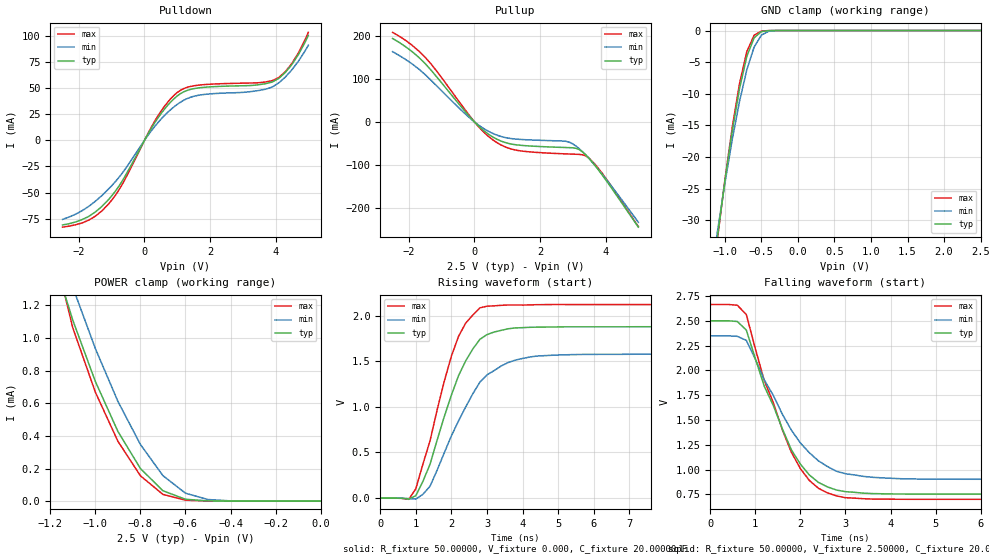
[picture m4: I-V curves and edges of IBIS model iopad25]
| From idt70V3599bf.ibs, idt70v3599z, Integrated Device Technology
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|   Model iopad25
[Model]   iopad25
Model_type   I/O
Polarity   Non-Inverting
Enable   Active-Low
Vinl =  0.70000V
Vinh =  1.70000V
Vmeas =  1.25000V
C_comp   4.50000pF   NA   NA
[Temperature Range]   25.00000   100.00000   0.000
[Voltage Range]   2.50000V   2.30000V   2.70000V
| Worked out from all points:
|   slope of the pulldown table from 0 to 0.375 V, typ, clamps not added: 19 ohm
|   slope of the pullup table from 0 to 0.375 V, typ, clamps not added: 14.7 ohm
|   GND clamp passes 1 mA (typ) near -0.58 V on its own axis
|   POWER clamp passes 1 mA (typ) near -1.07 V on its own axis
|   rising waveform, R_fixture 50.00000, V_fixture 0.000, C_fixture 20.00000pF: 20-80 % time 997ps typ, 1.18ns min, 891ps max; typ from 0 V to 1.88 V
|   falling waveform, R_fixture 50.00000, V_fixture 2.50000, C_fixture 20.00000pF: 20-80 % time 957ps typ, 1.1ns min, 930ps max; typ from 2.5 V to 0.752 V
[Pulldown]
| voltage   I(typ)   I(min)   I(max)
-2.5V     -80.9mA    -75.6mA    -83mA
-1.7V     -72.72mA   -63.11mA   -76.3mA
-1.1V     -56.75mA   -46.65mA   -61mA
-700mV    -39.93mA   -32.22mA   -43.24mA
400mV     20.93mA    16.57mA    22.86mA
1V        42.48mA    34.41mA    45.78mA
1.6V      49.93mA    42.82mA    52.59mA
3.2V      52.4mA     46.46mA    54.8mA
3.9V      55.8mA     51.01mA    57.1mA
4.1V      59.27mA    54.98mA    60.15mA
4.5V      72.61mA    67.54mA    73.61mA
5V        100.4mA    90.94mA    103.3mA
[Pullup]
| voltage   I(typ)   I(min)   I(max)
-2.5V     193.7mA    163.2mA    208mA
-1.9V     162.9mA    134.5mA    177.7mA
-1.5V     135.1mA    109.5mA    149.5mA
0V        0A         0A         0A
600mV     -36.73mA   -28.02mA   -43.74mA
900mV     -46.86mA   -35.51mA   -56.68mA
1.3V      -53.27mA   -39.97mA   -65.84mA
2.8V      -59.36mA   -45.06mA   -74.12mA
3.1V      -61.19mA   -56.09mA   -74.96mA
3.4V      -76.58mA   -76.99mA   -79.01mA
3.7V      -103mA     -102.7mA   -99.96mA
5V        -244.1mA   -232.8mA   -243mA
[GND_clamp]
| voltage   I(typ)   I(min)   I(max)
-2.5V     -180.9mA   -164.8mA   -186.8mA
-1.1V     -32.46mA   -31.63mA   -32.77mA
-1V       -23.79mA   -24.13mA   -23.62mA
-900mV    -15.93mA   -17.27mA   -15.36mA
-800mV    -9.216mA   -11.21mA   -8.395mA
-700mV    -4.104mA   -6.21mA    -3.33mA
-600mV    -1.149mA   -2.618mA   -751.2uA
-500mV    -171.6uA   -715.3uA   -87.25uA
-400mV    -15.64uA   -119.9uA   -6.065uA
-300mV    -924.1nA   -14.35uA   -255.2nA
2.5V      312.7pA    48.33nA    40.79pA
[POWER_clamp]
| voltage   I(typ)   I(min)   I(max)
-2.5V     38.57mA    31.01mA    47.82mA
-1.2V     1.551mA    1.733mA    1.63mA
-1.1V     1.109mA    1.311mA    1.062mA
-1V       734uA      935.8uA    668.2uA
-900mV    427.8uA    612uA      367.5uA
-800mV    200.1uA    347.7uA    155.6uA
-700mV    63.56uA    156.3uA    41.28uA
-600mV    11.54uA    48.7uA     5.887uA
-500mV    1.339uA    9.858uA    548.3nA
-400mV    116.5nA    1.522uA    36.02nA
0V        312.7pA    26.91nA    46.51pA
[Ramp]
| variable   typ   min   max
dV/dt_r   1.12740/0.44263n   0.94680/0.59313n   1.27380/0.36724n
dV/dt_f   1.05030/0.24636n   0.89232/0.28947n   1.16016/0.23207n
R_load = 50.00000
[Rising Waveform]
R_fixture = 50.00000
V_fixture = 0.000
C_fixture = 20.00000pF
R_dut = 100.00000m
L_dut = 4.00000nH
C_dut = 0.64000pF
| time   V(typ)   V(min)   V(max)
0s        0V         0V         0V
800ps     -10.49mV   -4.607mV   -13.1mV
1ns       27.07mV    -10.32mV   103.5mV
1.4ns     372.5mV    131.1mV    630mV
2ns       1.129V     682.7mV    1.556V
2.4ns     1.502V     997.2mV    1.917V
2.8ns     1.739V     1.27V      2.084V
3.6ns     1.855V     1.486V     2.115V
4.4ns     1.873V     1.556V     2.119V
10ns      1.877V     1.576V     2.12V
[Falling Waveform]
R_fixture = 50.00000
V_fixture = 2.50000
C_fixture = 20.00000pF
R_dut = 100.00000m
L_dut = 4.00000nH
C_dut = 0.64000pF
| time   V(typ)   V(min)   V(max)
0s        2.5V       2.348V     2.664V
600ps     2.493V     2.343V     2.657V
800ps     2.406V     2.302V     2.563V
1.2ns     1.838V     1.902V     1.894V
1.8ns     1.198V     1.397V     1.174V
2.2ns     944.1mV    1.169V     888.9mV
2.6ns     824.5mV    1.03V      764.3mV
3ns       776.5mV    957.1mV    715.5mV
4.2ns     753mV      907.4mV    700mV
10ns      751.7mV    901.3mV    699.2mV
